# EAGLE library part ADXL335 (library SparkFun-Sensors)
Analog Devices ADXL335 3-Axis Analog Accelerometer The ADXL335 is a small, thin, low power, complete 3-axis accelerometer with signal conditioned voltage outputs. The product measures acceleration with a minimum full-scale range of ±3 g. It can measure the static acceleration of gravity in tiltsensing applications, as well as dynamic acceleration resulting from motion, shock, or vibration. Datasheet SparkFun Products SparkFun Triple Axis Accelerometer Breakout - ADXL335 (SEN-09269) Triple Axis Accelerometer - ADXL335 (SEN-09265)
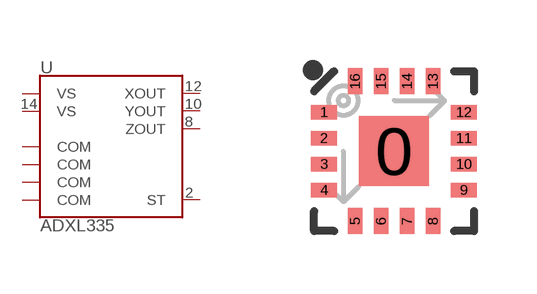
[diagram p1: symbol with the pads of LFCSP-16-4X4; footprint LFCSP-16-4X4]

Designator prefix U

## ADXL335 (PROD_ID: IC-08942; SF_ID: COM-09265)  [LFCSP-16-4X4]
2  ST
3  COM
5  COM
6  COM
7  COM
8  ZOUT
10  YOUT
12  XOUT
14  VS
15  VS

## Footprint LFCSP-16-4X4 (pad centres in mm)
16-Pin LFCSP w/ Center Pad (4 x 4 mm) Datasheet Specifications: Pin Count: 16 (+ center pad) Area: 4.0 x 4.0 x 1.45 mm Pitch: 0.65 mm Devices Using: ADXL330 ADXL335
smd 1.75 x 1.75: 0 0,0
smd 0.65 x 0.37: 1 -1.75,0.975; 2 -1.75,0.325; 3 -1.75,-0.325; 4 -1.75,-0.975; 9 1.75,-0.975; 10 1.75,-0.325; 11 1.75,0.325; 12 1.75,0.975
smd 0.37 x 0.65: 5 -0.975,-1.75; 6 -0.325,-1.75; 7 0.325,-1.75; 8 0.975,-1.75; 13 0.975,1.75; 14 0.325,1.75; 15 -0.325,1.75; 16 -0.975,1.75

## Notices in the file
Licensing: Creative Commons ShareAlike 4.0 International - https://creativecommons.org/licenses/by-sa/4.0
